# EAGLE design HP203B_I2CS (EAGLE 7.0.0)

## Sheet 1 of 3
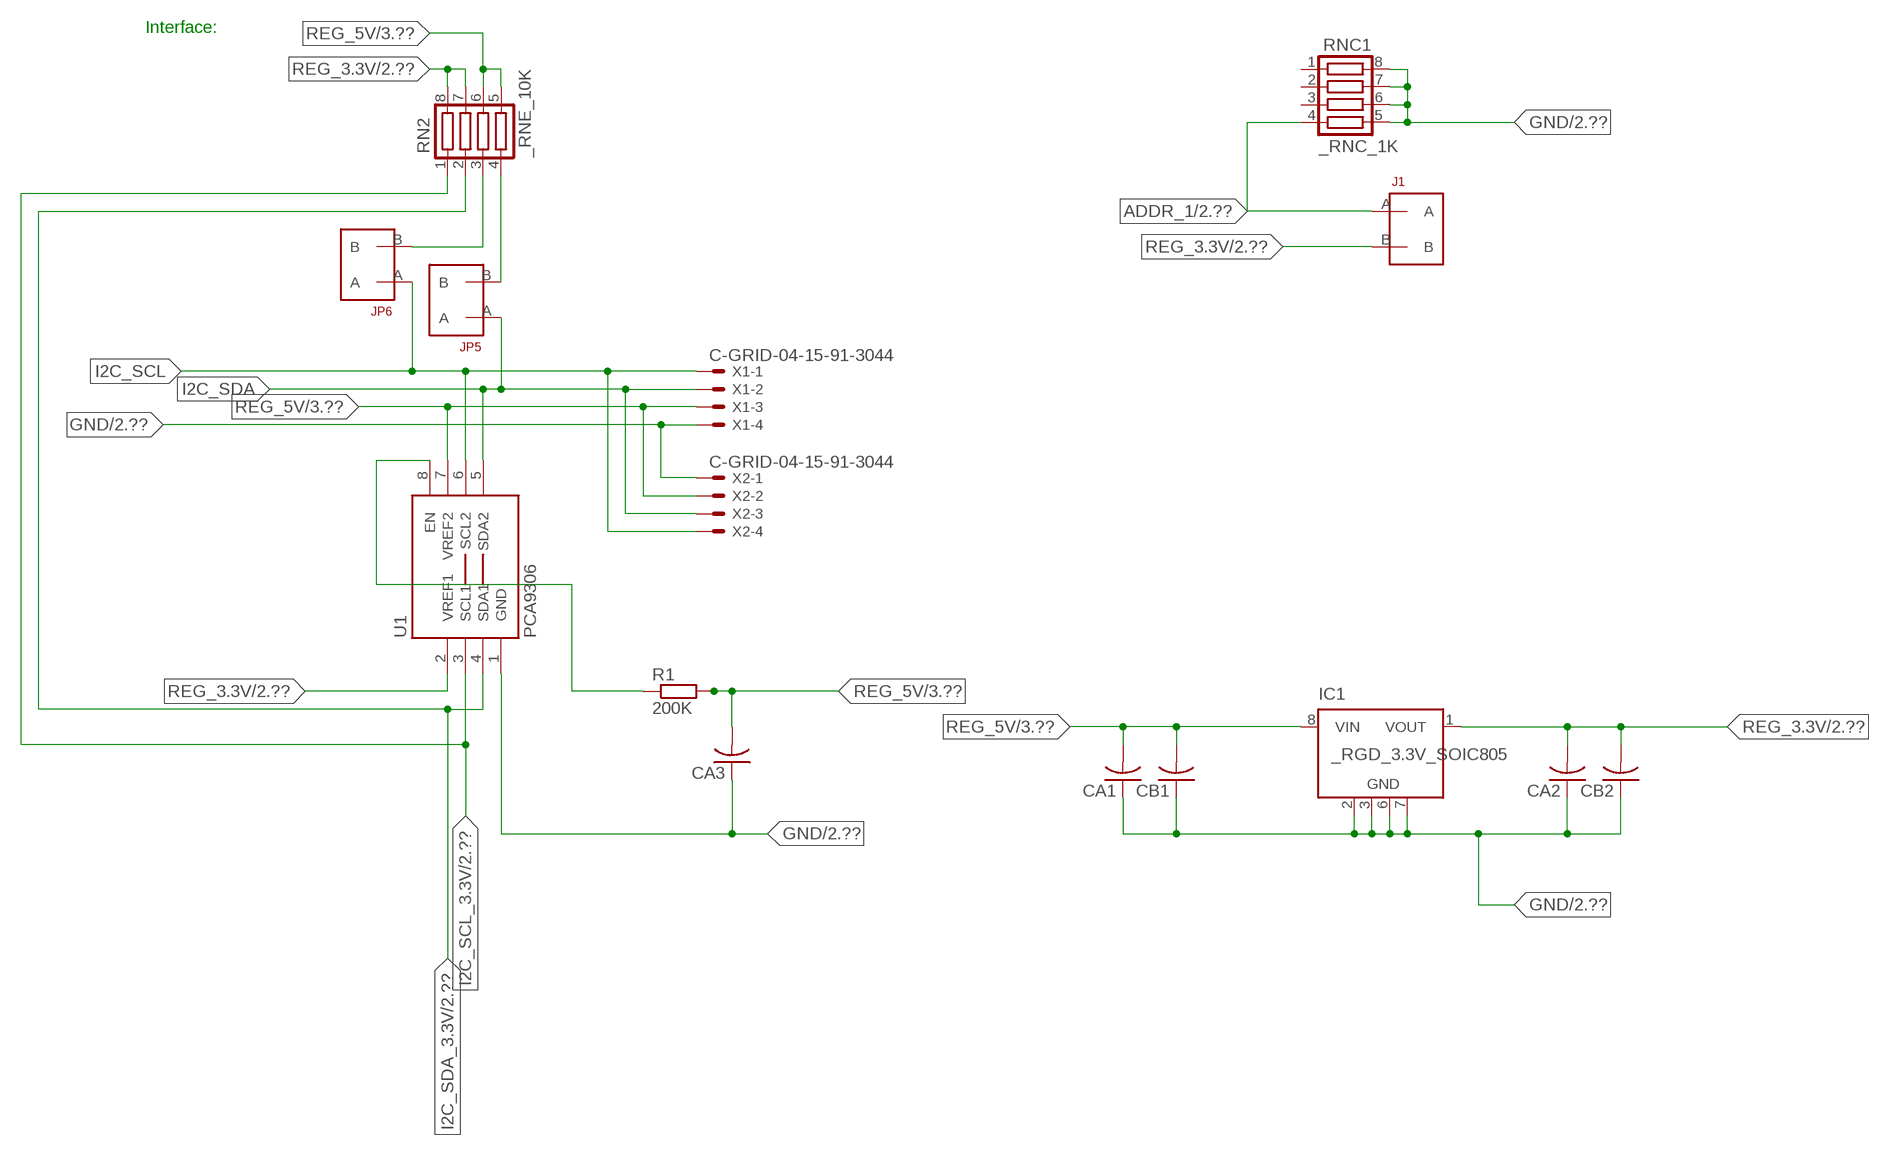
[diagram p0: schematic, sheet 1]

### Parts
CA1  CC1206KRX7R9BB104  [.1UF]
CA2  CC1206KRX7R9BB104  [.1UF]
CA3  CC1206KRX7R9BB104  [.1UF]
CB1  TMK316F106ZL-TC1206K  [TMK316F106ZL-T]
CB2  TMK316F106ZL-TC1206K  [TMK316F106ZL-T]
IC1  _RGD_3.3V_SOIC805  [_RGC_3.3V_SOIC8]
J1  JUMPER_1X2_2MM  [JUMPER_1X2_2MM]
JP5  JUMPER_1X2_2MM  [JUMPER_1X2_2MM]
JP6  JUMPER_1X2_2MM  [JUMPER_1X2_2MM]
R1  200K  RESISTOR_SMT-0603  [R603]
RN2  _RNE_10K  [RNE]
RNC1  _RNC_1K  [RNC]
U1  PCA9306  PCA9306_NCD  [PSOP-8]
X1  C-GRID-04-15-91-3044  [15-91-04]
X2  C-GRID-04-15-91-3044  [15-91-04]

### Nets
ADDR_1: J1.A RNC1.4 ; also sheet 2
GND: CA1.1 CA2.1 CA3.1 CB1.1 CB2.1 IC1.2(GND) IC1.3(GND) IC1.6(GND) IC1.7(GND) RNC1.5 RNC1.6 RNC1.7 RNC1.8 U1.1(GND) X1.4 X2.1 ; also sheet 2,3
I2C_SCL: JP6.A U1.6(SCL2) X1.1 X2.4
I2C_SCL_3.3V: RN2.1 U1.3(SCL1) ; also sheet 2
I2C_SDA: JP5.A U1.5(SDA2) X1.2 X2.3
I2C_SDA_3.3V: RN2.2 U1.4(SDA1) ; also sheet 2
N$1: JP6.B RN2.3
N$2: JP5.B RN2.4
N$3: R1.1 U1.8(EN)
REG_3.3V: CA2.2 CB2.2 IC1.1(VOUT) J1.B RN2.7 RN2.8 U1.2(VREF1) ; also sheet 2
REG_5V: CA1.2 CA3.2 CB1.2 IC1.8(VIN) R1.2 RN2.5 RN2.6 U1.7(VREF2) X1.3 X2.2 ; also sheet 3
Unconnected: IC1.4(NC) IC1.5(NC) RNC1.1 RNC1.2 RNC1.3

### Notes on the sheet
- Interface:

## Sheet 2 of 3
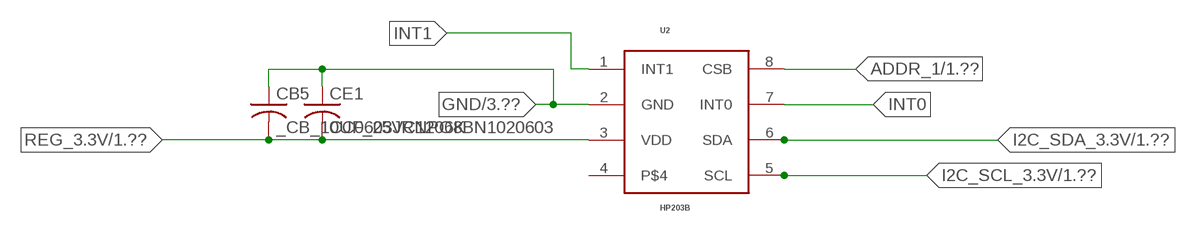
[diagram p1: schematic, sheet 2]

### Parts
CB5  _CB_10UF_25VC1206K  [_CB_10UF_25V]
CE1  CC0603JRNPO8BN1020603  [CC0603JRNPO8BN102]
U2  HP203B  [HP203]

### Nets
ADDR_1: U2.8(CSB) ; also sheet 1
GND: CB5.1 CE1.1 U2.2(GND) ; also sheet 1,3
I2C_SCL_3.3V: U2.5(SCL) ; also sheet 1
I2C_SDA_3.3V: U2.6(SDA) ; also sheet 1
INT0: U2.7(INT0)
INT1: U2.1(INT1)
REG_3.3V: CB5.2 CE1.2 U2.3(VDD) ; also sheet 1
Unconnected: U2.4

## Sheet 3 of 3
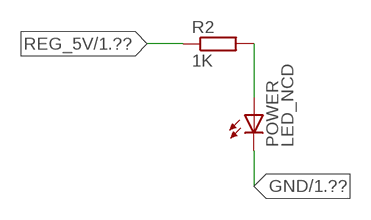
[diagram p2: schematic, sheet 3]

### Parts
POWER  LED_NCD  [CHIPLED_0603]
R2  1K  RESISTOR_SMT-0402  [R402]

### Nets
GND: POWER.C ; also sheet 1,2
N$4: POWER.A R2.2
REG_5V: R2.1 ; also sheet 1

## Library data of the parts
CA1-CA3 = NCD_ULTIMATE_LIBRARY:CC1206KRX7R9BB104: Capacitor CA .1uF 50V SMT C1206K CC1206KRX7R9BB104
CB1 CB2 = NCD_ULTIMATE_LIBRARY:TMK316F106ZL-T: Capacitor CB 10uF SMT 1206 TMK316F106ZL-T
CB5 = NCD_ULTIMATE_LIBRARY:_CB_10UF_25V: Capacitor 10uF SMT
CE1 = NCD_ULTIMATE_LIBRARY:CC0603JRNPO8BN102: Capacitor CE 1uF SMT CC0603JRNPO8BN102 0603
IC1 = NCD_ULTIMATE_LIBRARY:_RGD_3.3V_SOIC8: Regulator Linear 3.3V Chip Positive VOLTAGE REGULATOR Digikey 497-1199-2-ND/L78L33ACD13TR
J1 JP5 JP6 = NCD_ULTIMATE_CONNECTORS:JUMPER_1X2_2MM
POWER = NCD_ULTIMATE_LIBRARY:LED_NCD: LED Digikey 754-1132-2-ND/APT2012SRCPRV
R1 R2 = NCD_ULTIMATE_LIBRARY:RESISTOR_SMT: NCD Resistor
RN2 = NCD_ULTIMATE_LIBRARY:_RNE_10K: Resistor Array RNE SMT 10K x 4 Single Resistor Source: http://www.ctscorp.com/components/Datasheets/CTSChipArrayDs.pdf Digikey 742C083103JPTR-ND/742C083103JP; OC_FARNELL: unknown; OC_NEWARK: unknown
RNC1 = NCD_ULTIMATE_LIBRARY:_RNC_1K: Resistor Array RNC SMT 1K x 4 Single Resistor Source: http://www.ctscorp.com/components/Datasheets/CTSChipArrayDs.pdf Digikey 742C083102JPTR-ND/742C083102JP; OC_FARNELL: unknown; OC_NEWARK: unknown
U1 = NCD_ULTIMATE_LIBRARY:PCA9306_NCD: NCD Bidirectional I2C level shifter. NOT compatible with all available part number pinout schemes- DOUBLE CHECK!!!; PROD_ID: IC-10023
U2 = NCD_ULTIMATE_bhaskar:HP203B
X1 X2 = NCD_ULTIMATE_CONNECTORS:C-GRID-04: CONNECTOR 4-Pos I2C wire to board 2.54 mm (0.100") pitch header Digikey WM1342-ND/0015912045; OC_FARNELL: unknown; OC_NEWARK: unknown

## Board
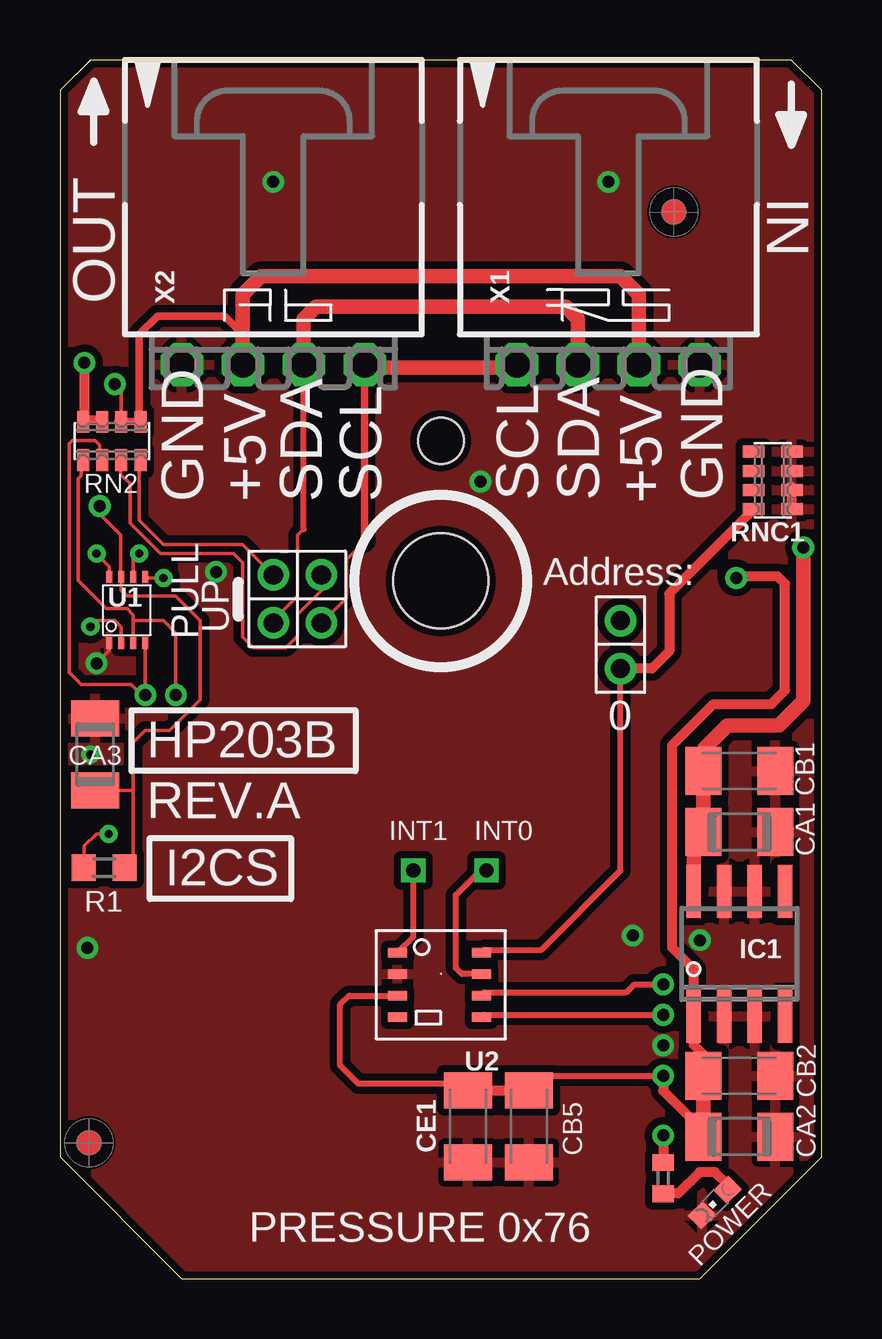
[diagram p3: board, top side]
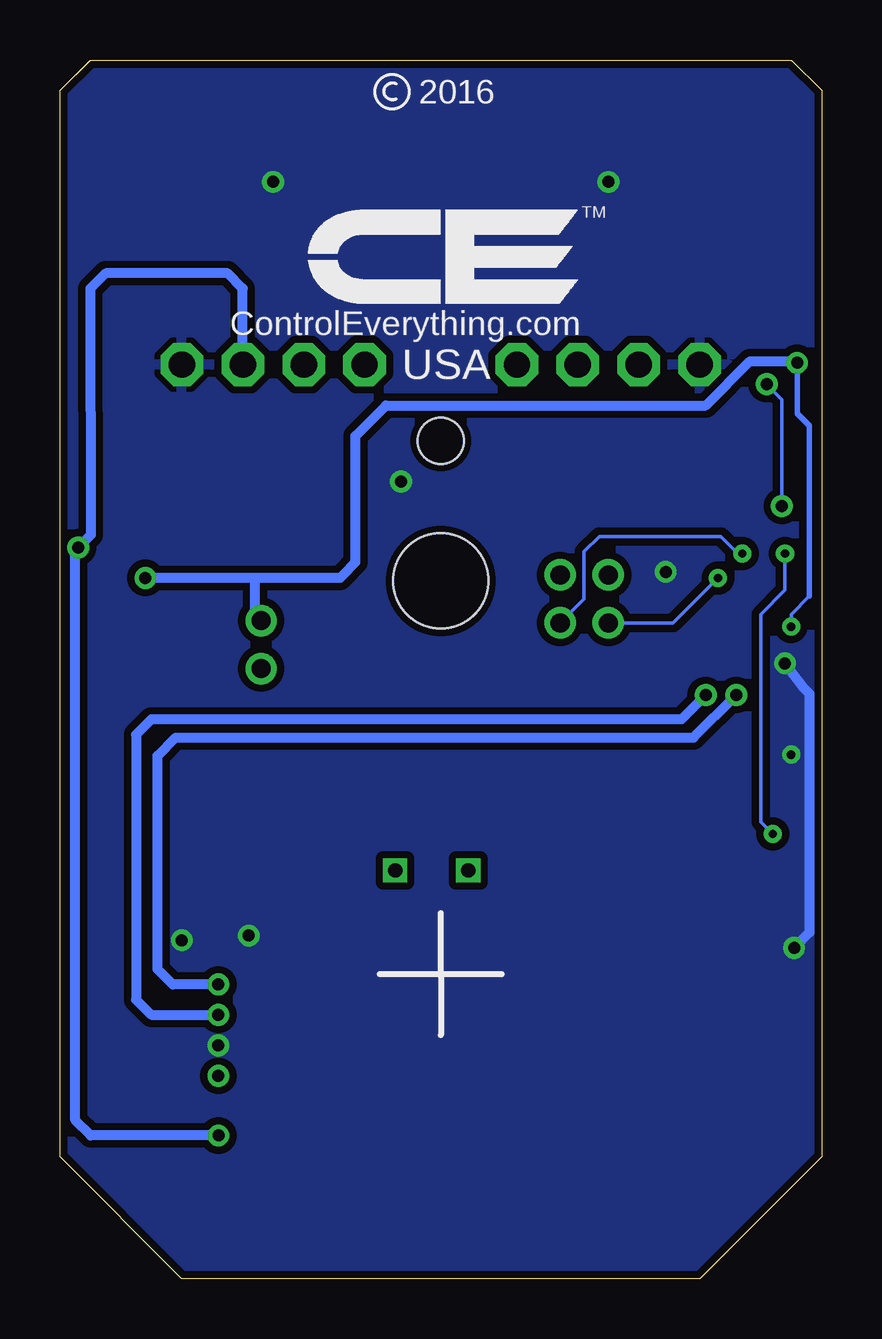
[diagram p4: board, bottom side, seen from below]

Size 31.75 x 50.8 mm. Coordinates in mm from the lower left corner, seen from the top.
Outline: 31.75,5.08 31.75,49.53 30.48,50.8 1.27,50.8 0,49.53 0,5.08 5.08,0 26.67,0 31.75,5.08
Outline: 31.75,5.08 31.75,49.53 30.48,50.8 1.27,50.8 0,49.53 0,5.08 5.08,0 26.67,0 31.75,5.08
Copper layers (1*16): Top 0.035mm / dielectric 1.5mm / Bottom 0.035mm
Design rules "default": minimum track width 5mil, minimum drill 24mil, track to track 5mil, track to pad 5mil, pad to pad 5mil, via to via 5mil, smd to smd 5mil, copper to edge 10mil, drill to drill 8mil, minimum pad ring 10mil, minimum via ring 8mil, stop-mask expansion 2mil, vias tented up to drill 0mil, thermal gap 10mil
Holes 3.96 mm at 15.88,29.08
Holes 1.91 mm at 15.88,34.93

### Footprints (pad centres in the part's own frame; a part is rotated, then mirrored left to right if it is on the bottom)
.1UF = smd 1.5 x 2: 1 -1.5,0; 2 1.5,0
TMK316F106ZL-T = smd 1.5 x 2: 1 -1.5,0; 2 1.5,0
_CB_10UF_25V = smd 1.5 x 2: 1 -1.5,0; 2 1.5,0
CC0603JRNPO8BN102 = smd 1.5 x 2: 1 -1.5,0; 2 1.5,0
_RGC_3.3V_SOIC8 = smd 0.6 x 2.2: 1 -1.905,-2.6; 2 -0.635,-2.6; 3 0.635,-2.6; 4 1.905,-2.6; 5 1.905,2.6; 6 0.635,2.6; 7 -0.635,2.6; 8 -1.905,2.6
JUMPER_1X2_2MM = drill 0.8: A 0,2; B 0,0
CHIPLED_0603 = smd 0.8 x 0.876: A 0,-0.75; C 0,0.75
R603 = smd 1 x 1.1: 1 -0.85,0; 2 0.85,0
R402 = smd 0.7 x 0.9: 1 -0.65,0; 2 0.65,0
RNE = smd 0.5 x 0.9: 1 -1.2,-0.8; 2 -0.4,-0.8; 3 0.4,-0.8; 4 1.2,-0.8; 5 1.2,0.8; 6 0.4,0.8; 7 -0.4,0.8; 8 -1.2,0.8
RNC = smd 0.5 x 0.9: 1 -1.2,-0.8; 2 -0.4,-0.8; 3 0.4,-0.8; 4 1.2,-0.8; 5 1.2,0.8; 6 0.4,0.8; 7 -0.4,0.8; 8 -1.2,0.8
PSOP-8 = smd 0.25 x 0.5: 1 -0.73,-1.37; 2 -0.23,-1.37; 3 0.27,-1.37; 4 0.77,-1.37; 5 0.77,1.38; 6 0.27,1.38; 7 -0.23,1.38; 8 -0.73,1.38
HP203 = smd 0.4 x 0.8: 1 -0.9,-1.8; 2 0,-1.8; 3 0.9,-1.8; 4 1.8,-1.8; 5 1.8,1.7; 6 0.9,1.7; 7 0,1.7; 8 -0.9,1.7
15-91-04 = drill 1.1 pad 1.778 octagon: 1 -3.81,-7.62; 2 -1.27,-7.62; 3 1.27,-7.62; 4 3.81,-7.62

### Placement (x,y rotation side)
CA1  28.32,18.62 180 top
CA2  28.32,5.92 180 top
CA3  1.46,21.86 270 top
CB1  28.32,21.16 180 top
CB2  28.32,8.46 180 top
CB5  19.56,6.35 90 top
CE1  17.02,6.35 90 top
IC1  28.32,13.54 0 top
J1  23.37,27.43 180 top
JP5  8.89,29.34 180 top
JP6  10.9,29.34 180 top
POWER  27.3,3.18 135 top
R1  1.84,17.13 0 top
R2  25.15,4.19 270 top
RN2  2.16,34.93 0 top
RNC1  29.72,33.27 270 top
U1  2.79,27.86 0 top
U2  15.88,12.7 270 top
U$5  [VISION_REF10]  1.21,5.66 90 top
U$28  [VISION_REF10]  25.59,44.46 90 top
X1  22.86,45.72 0 top
X2  8.89,45.72 0 top

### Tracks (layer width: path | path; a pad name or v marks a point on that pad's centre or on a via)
ADDR_1
  Top 0.254: U2.8 17.69,13.72 20.07,13.72 23.37,17.02 J1.A
  Top 0.406: RNC1.4 25.4,28.56 25.4,26.16 24.67,25.43 J1.A
GND  (via drill 0.35, 0.5)
  Top 0.152: CA3.1 1.52,23.42 1.52,23.62 | v1.52,25.65 2.06,26.19 U1.1
  Top 0.406: RNC1.5 30.52,32.98 30.48,33.02
  Bottom 0.406: v1.52,25.65 0.76,24.64 0.51,24.38 0.51,14.43 v1.15,13.79
  other vias: 8.89,45.72 22.86,45.72 25.15,9.73 17.53,33.22 26.67,14.11 6.5,29.46 1.27,21.84 23.88,14.3
  pour Bottom (isolate 0.305): -0.64,5.08 -0.64,49.53 1.27,51.44 30.48,51.44 32.38,49.53 32.38,5.08 26.67,-0.63 5.08,-0.63
  pour Top (isolate 0.305): 4.45,-1.27 -1.27,4.45 -1.27,50.17 0.64,52.07 31.11,52.07 33.02,50.17 33.02,4.45 27.3,-1.27
I2C_SCL  (via drill 0.35)
  Top 0.152: 12.7,30.73 11.94,29.97 11.94,28.38 JP6.A | v3.3,30.23 3.06,29.99 U1.6
  Top 0.305: 12.7,30.73 X2.4
  Top 0.406: X2.4 12.7,37.97 | 19.05,37.97 X1.1
  Top 0.61: 12.7,37.97 19.05,37.97
  Bottom 0.152: JP6.A 9.91,28.33 9.91,30.3 9.27,30.94 4.19,30.94 3.48,30.23 v3.3,30.23
I2C_SCL_3.3V  (via drill 0.5)
  Top 0.152: RN2.1 0.89,34.07 0.89,33.48 0.77,33.35 0.77,29.1 1.92,27.94 2.79,27.94 3.06,27.67 3.06,27.43 | 3.06,27.43 U1.3 | v4.83,24.33 v4.83,24.34 4.83,26.92 4.32,27.43 3.06,27.43
  Top 0.254: U2.5 17.67,11 v25.15,11
  Bottom 0.406: v4.83,24.33 5.84,23.32 27.94,23.32 28.58,22.68 28.58,11.63 27.94,11 v25.15,11
I2C_SDA  (via drill 0.35)
  Top 0.152: JP5.A 8.89,27.44 9.91,28.45 9.91,30.99 10.16,31.24 | U1.5 3.6,29.21 v4.32,29.21
  Top 0.254: 10.16,31.24 10.16,31.25 X2.3
  Top 0.61: X2.3 10.16,40.01 10.67,40.51 21.09,40.51 21.59,40.01 X1.2
  Bottom 0.152: v4.32,29.21 6.19,27.34 JP5.A
I2C_SDA_3.3V  (via drill 0.5)
  Top 0.152: RN2.2 1.65,34.14 1.65,34.75 1.46,34.94 0.51,34.94 0.38,34.81 0.38,26.37 0.38,26.36 0.38,25.27 0.89,24.77 2.97,24.77 3.4,24.33 v3.56,24.33 v3.56,24.34 U1.4
  Top 0.254: U2.6 17.71,11.94 23.62,11.94 23.95,12.27 v25.15,12.27
  Top 0.406: 25.07,12.27 v25.15,12.27
  Bottom 0.406: v25.15,12.27 27.05,12.27 27.69,12.9 27.69,21.79 26.93,22.56 5.34,22.56 v3.56,24.33
INT0  (via drill 0.6)
  Top 0.254: U2.7 16.76,12.7 16.51,12.95 16.51,16 17.53,17.02 v17.78,17.02
INT1  (via drill 0.6)
  Top 0.254: U2.1 14.73,14.26 v14.73,17.02
N$1
  Top 0.152: JP6.B 10.92,29.31 10.92,28.7 9.91,27.69 9.91,26.8 9.42,26.31 8.06,26.31 7.62,26.75 7.62,29.84 7.24,30.23 4.19,30.23 2.92,31.5 2.92,33.15 2.54,33.53 2.54,34.1 RN2.3
  Top 0.305: 2.54,34.02 RN2.3
N$2
  Top 0.152: JP5.B 7.62,30.61 4.32,30.61 3.3,31.62 3.3,34.07 RN2.4
  Top 0.305: 3.37,33.88 RN2.4
N$3  (via drill 0.35)
  Top 0.152: R1.1 1.02,17.16 1.02,18.03 1.52,18.54 v2.03,18.54 | v1.52,30.23 2.06,29.69 U1.8
  Bottom 0.152: v2.03,18.54 2.54,19.05 2.54,27.69 1.52,28.7 v1.52,30.23
N$4
  Top 0.406: POWER.A 27.84,3.92 27.3,4.45 26.67,4.45 25.78,3.56 25.16,3.56 R2.2
REG_3.3V  (via drill 0.35, 0.5)
  Top 0.152: v1.27,27.18 1.52,27.43 2.29,27.43 2.56,27.16 U1.2
  Top 0.254: CB5.2 20.17,8.46 v25.15,8.46 | CE1.2 16.74,8.13 12.45,8.13 11.68,8.89 11.68,11.43 12.05,11.8 U2.3
  Top 0.406: CB2.2 26.82,9.35 26.42,9.75 26.42,10.36 | v25.15,8.46 25.15,7.82 26.42,6.55 26.82,6.55 | IC1.1 26.42,12.9 25.53,13.79 25.53,22.24 27.24,23.95 29.66,23.95 30.23,24.52 30.23,28.97 29.91,29.29 28.27,29.29 v28.19,29.21 | 26.52,5.62 CA2.2 | v1.02,38.18 1.02,35.78 | 1.02,35.78 RN2.8 | 1.02,35.78 1.71,35.78 RN2.7 | CE1.2 CB5.2
  Top 0.61: CB2.2 26.82,6.55 CA2.2 | 26.42,10.36 IC1.1
  Bottom 0.152: 0.51,28.45 1.27,27.69 v1.27,27.18
  Bottom 0.229: 0.51,28.45 0.51,35.56 1.02,36.07 v1.02,38.18
  Bottom 0.406: v1.02,38.18 1.08,38.24 2.99,38.24 4.83,36.4 18.16,36.4 19.43,35.13 19.43,29.87 19.94,29.34 20.07,29.21 23.62,29.21 | 23.62,29.21 v28.19,29.21 | J1.B 23.62,27.69 23.62,29.21
REG_5V  (via drill 0.5)
  Top 0.152: RN2.6 2.56,37.01 v2.29,37.29 | R1.2 3.05,17.49 3.05,20.36 | 3.05,20.36 3.05,22.35 3.56,22.86 4.57,22.86 5.84,24.13 5.84,27.43 4.83,28.45 2.79,28.45 2.56,28.68 U1.7 2.54,29.27 2.54,30.99 1.65,31.87 v1.65,32.21 | CA3.2 3.05,20.36
  Top 0.305: 7.62,39.37 7.5,39.37 | 2.42,35.74 RN2.6 RN2.5 3.31,35.8 3.31,39.37 4.07,40.13 6.86,40.13 7.62,39.37 | X2.2 7.62,39.37
  Top 0.406: v25.15,5.97 R2.1
  Top 0.61: X2.2 7.62,41.02 8.38,41.78 23.37,41.78 24.13,41.02 X1.3 | IC1.8 26.42,18.21 CA1.2 CB1.2 26.86,21.2 26.86,22.11 27.82,23.06 29.98,23.06 30.99,24.08 v30.99,30.48
  Bottom 0.152: v1.65,32.21 1.65,36.65 v2.29,37.29
  Bottom 0.406: X1.3 24.13,41.28 24.77,41.91 29.84,41.91 30.48,41.27 30.47,31 v30.99,30.48 31.11,30.36 31.11,6.6 30.48,5.97 v25.15,5.97

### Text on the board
tNames: IN | OUT | GND | +5V | SDA | SCL | SCL | SDA | +5V | GND | Address: | PULL | UP | 0 | HP203B | REV.A | INT1 | INT0 | I2CS | PRESSURE 0x76
bNames: 2016 | TM | ControlEverything.com | USA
